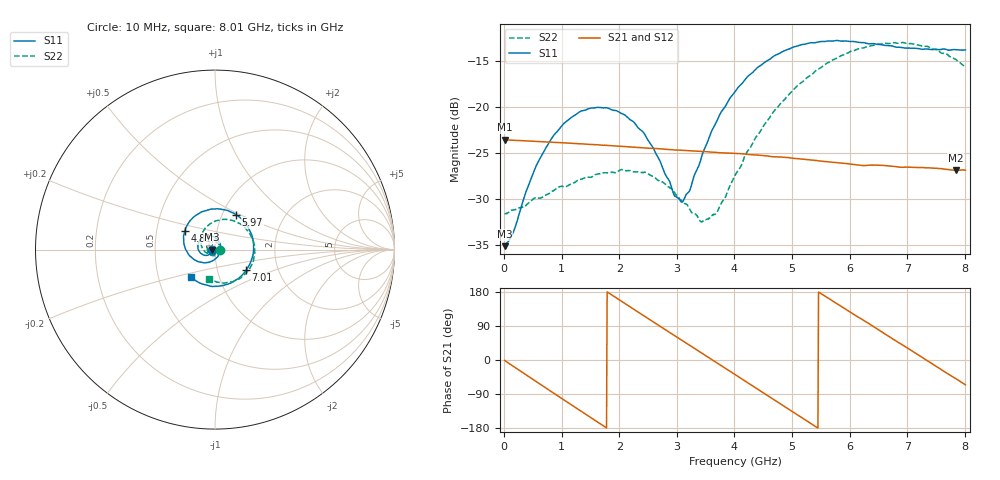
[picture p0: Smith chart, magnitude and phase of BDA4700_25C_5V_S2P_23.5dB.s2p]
!Agilent Technologies,E5071B,MY42404982,A.09.10
!Date: Mon Oct 20 13:38:15 2025
!Data & Calibration Information:
!Freq	S11:SOLT2(ON)	S21:SOLT2(ON)	S12:SOLT2(ON)	S22:SOLT2(ON)
# Hz S RI R 50
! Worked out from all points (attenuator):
!   801 points, 10 MHz to 8.01 GHz, reference 50 ohm
!   highest |S21| = -23.58 dB at 10 MHz (marker M1); lowest = -26.9 dB at 7.84 GHz (marker M2)
!   lowest |S11| = -35.2 dB at 10 MHz (marker M3), VSWR 1.04, Z = 48.3 - j0.0997 ohm
!   |S11| at or under -10 dB: start of sweep to end of sweep
!   |S22| runs from -32.5 to -13.0 dB; largest |S21 - S12| = 0.00055
!   S11 on the Smith chart (normalised r, x): 10 MHz: 0.97, -0.00; 4.81 GHz: 0.70, +0.15; 5.97 GHz: 1.16, +0.48; 7.01 GHz: 1.37, -0.33; 8.01 GHz: 0.73, -0.24
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1e7  -0.0174 -0.00103  0.0662 -0.00143  0.0662 -0.00146  0.0262 -0.00083
1.6e8  -0.0183 -0.00968  0.063 -0.0188  0.063 -0.0188  0.0264 -0.00753
5.1e8  -0.0335 -0.0282  0.0399 -0.0512  0.0399 -0.0512  0.0168 -0.0266
7.3e8  -0.0506 -0.0322  0.0175 -0.062  0.0174 -0.0619  0.00383 -0.033
1.35e9  -0.0949 0.00542  -0.0454 -0.0433  -0.0455 -0.0433  -0.0364 -0.0177
2.09e9  -0.0506 0.0749  -0.0526 0.0304  -0.0526 0.0304  -0.029 0.0346
2.42e9  -0.00777 0.072  -0.0275 0.0531  -0.0275 0.0531  -0.00431 0.0436
2.68e9  0.0193 0.049  -0.00191 0.0591  -0.00191 0.059  0.0136 0.0373
2.96e9  0.031 0.0107  0.0251 0.0525  0.0251 0.0524  0.026 0.0222
3.1e9  0.0286 -0.01  0.0367 0.0448  0.0366 0.0449  0.0284 0.0109
3.41e9  0.0023 -0.0506  0.0536 0.02  0.0537 0.02  0.0204 -0.0124
3.54e9  -0.0157 -0.0632  0.0564 0.0076  0.0564 0.0075  0.0127 -0.021
3.7e9  -0.0441 -0.0716  0.0558 -0.00775  0.0558 -0.00794  -0.00112 -0.0267
4.01e9  -0.1034 -0.062  0.0437 -0.0346  0.0438 -0.0345  -0.033 -0.0262
4.81e9  -0.1687 0.1022  -0.0241 -0.0475  -0.024 -0.0475  -0.0786 0.0695
5.35e9  -0.0695 0.2118  -0.0505 -0.009  -0.0504 -0.00921  -0.0152 0.1491
5.97e9  0.1178 0.1941  -0.0315 0.0375  -0.0317 0.0374  0.1254 0.1504
6.68e9  0.2144 -0.0113  0.0221 0.0422  0.0223 0.0422  0.2207 -0.00181
7.01e9  0.1733 -0.1157  0.0402 0.0243  0.0403 0.024  0.2012 -0.0902
7.45e9  0.0485 -0.1991  0.0454 -0.00933  0.0454 -0.00949  0.1116 -0.1723
7.84e9  -0.083 -0.1867  0.0296 -0.0341  0.0297 -0.0341  0.0089 -0.181
8.01e9  -0.132 -0.1552  0.0187 -0.0411  0.0188 -0.0411  -0.0325 -0.1612
